| TEXAS INSTRUMENTS INCORPORATED
| Standard Linear and Logic Group
| IBIS Model of SN74ALVC245
| OCTAL BUS TRANSCEIVER WITH 3-STATE OUTPUTS
| This file contains package information for the following:
|  TVSOP 20-pin (DGV) package as [Component] ALVC245_DGV
|  SOIC 20-pin (DW) package as [Component] ALVC245_DW
|  SOP 20-pin (NS) package as [Component] ALVC245_NS
|  TSSOP 20-pin (PW) package as [Component] ALVC245_PW
|  QFN 20-pin (RGY) package as [Component] ALVC245_RGY
| This device can be powered at the following Vccs:
|  1.8 volt Vcc
|  2.5 volt Vcc
|  3.3 volt Vcc
| This file provides unique models under the [Model Selector] for each Vcc.
| For operation at a specific Vcc, select the appropriate model after each
| [Model Selector] keyword.
[IBIS Ver]   3.2
[Comment char]  |_char
[File Name]   sn74alvc245.ibs
[File Rev]   1.2 | d_die
[Date]   September 17, 2003
[Source]   Data created from TI-SPICE simulations at TI-SLL.
[Notes]   The following is an IBIS list for the SN74ALVC245.
   Please contact sllibis@ti.com with questions and
   comments concerning SLL IBIS models.
   - We removed Power_Clamp curve from the input models
   since there is no power clamp diode there.
   - Non-monotonic data in pulldown due to device characteristics.
[Disclaimer] Property of Texas Instruments Incorporated.  Unauthorized
   reproduction and/or distribution is strictly prohibited.
   This product is protected under copyright law.
   Created  2002, (C) Copyright  2002, Texas Instruments
   Incorporated, All Rights Reserved
   UNLESS THERE IS A SIGNED, WRITTEN AGREEMENT TO THE
   CONTRARY, TEXAS INSTRUMENTS (TI) IS PROVIDING THE IBIS
   MODELS  AND WITHOUT ANY WARRANTY, EXPRESSED OR
   IMPLIED.  TI assumes no liability for:
   1) the accuracy of the IBIS models provided to your
   company;
   2) the proper functioning of these IBIS Models in your
   design or for any resulting applications; or
   3) infringement of patents, copyrights or intellectual
   property rights resulting from your use of these IBIS
   models.
   TI provides IBIS Models as a service to our customers.
   You and your company shall not distribute, sell or give
   these models to anyone else without prior written
   permission from TI.
   TI reserves the right to make changes to our products or
   to discontinue any semiconductor product or service
   without notice, and advises our customers to obtain the
   latest version of relevant information to verify, before
   placing orders, that the information being relied on is
   current.
   Please be aware that your receipt and use of the IBIS
   information provided shall serve as acceptance of these
   terms and conditions.  If you do not accept these terms,
   you should return or destroy the IBIS models and any
   other accompanying information immediately.
| Component ALVC245_DGV 20-pin TVSOP
[Component]   ALVC245_DGV
[Manufacturer]  Texas Instruments, Inc.
[Package]
|   typ   min   max
R_pkg   4.400e-02   3.800e-02   4.800e-02
L_pkg   2.561e-09   2.236e-09   2.961e-09
C_pkg   3.420e-13   2.640e-13   4.460e-13
[Pin]   signal_name   model_name   R_pin   L_pin   C_pin
1   DIR   ALVC245_DIR   4.400e-02   2.935e-09   4.170e-13
2   A1   ALVC245_IO   4.200e-02   2.869e-09   4.460e-13
3   A2   ALVC245_IO   4.300e-02   2.399e-09   3.160e-13
4   A3   ALVC245_IO   4.400e-02   2.236e-09   2.650e-13
5   A4   ALVC245_IO   4.600e-02   2.278e-09   2.640e-13
6   A5   ALVC245_IO   4.500e-02   2.274e-09   2.640e-13
7   A6   ALVC245_IO   4.400e-02   2.285e-09   2.690e-13
8   A7   ALVC245_IO   4.300e-02   2.452e-09   3.200e-13
9   A8   ALVC245_IO   4.400e-02   2.900e-09   4.460e-13
10   GND   GND   4.400e-02   2.961e-09   4.180e-13
11   B8   ALVC245_IO   4.500e-02   2.954e-09   4.180e-13
12   B7   ALVC245_IO   4.200e-02   2.847e-09   4.430e-13
13   B6   ALVC245_IO   4.500e-02   2.453e-09   3.190e-13
14   B5   ALVC245_IO   4.500e-02   2.297e-09   2.690e-13
15   B4   ALVC245_IO   4.800e-02   2.334e-09   2.680e-13
16   B3   ALVC245_IO   4.800e-02   2.335e-09   2.670e-13
17   B2   ALVC245_IO   4.600e-02   2.299e-09   2.680e-13
18   B1   ALVC245_IO   4.600e-02   2.457e-09   3.200e-13
19   NOE   ALVC245_OE   4.300e-02   2.848e-09   4.410e-13
20   VCC   POWER   3.800e-02   2.812e-09   4.080e-13
| Component ALVC245_DW 20-pin SOIC
[Component]   ALVC245_DW
[Manufacturer]  Texas Instruments, Inc.
[Package]
|   typ   min   max
R_pkg   3.800e-02   3.300e-02   4.500e-02
L_pkg   5.012e-09   4.110e-09   6.349e-09
C_pkg   7.170e-13   5.300e-13   8.680e-13
[Pin]   signal_name   model_name   R_pin   L_pin   C_pin
1   DIR   ALVC245_DIR   4.200e-02   6.336e-09   8.650e-13
2   A1   ALVC245_IO   4.300e-02   5.542e-09   8.670e-13
3   A2   ALVC245_IO   3.400e-02   4.714e-09   7.320e-13
4   A3   ALVC245_IO   3.400e-02   4.377e-09   5.910e-13
5   A4   ALVC245_IO   3.600e-02   4.130e-09   5.330e-13
6   A5   ALVC245_IO   3.500e-02   4.111e-09   5.300e-13
7   A6   ALVC245_IO   3.400e-02   4.284e-09   5.830e-13
8   A7   ALVC245_IO   3.400e-02   4.634e-09   7.260e-13
9   A8   ALVC245_IO   4.000e-02   5.518e-09   8.650e-13
10   GND   GND   4.300e-02   6.349e-09   8.660e-13
11   B8   ALVC245_IO   4.100e-02   6.281e-09   8.610e-13
12   B7   ALVC245_IO   4.500e-02   5.561e-09   8.680e-13
13   B6   ALVC245_IO   3.300e-02   4.778e-09   7.420e-13
14   B5   ALVC245_IO   3.500e-02   4.414e-09   5.960e-13
15   B4   ALVC245_IO   3.500e-02   4.110e-09   5.330e-13
16   B3   ALVC245_IO   3.600e-02   4.130e-09   5.330e-13
17   B2   ALVC245_IO   3.400e-02   4.377e-09   5.910e-13
18   B1   ALVC245_IO   3.400e-02   4.714e-09   7.310e-13
19   NOE   ALVC245_OE   4.300e-02   5.569e-09   8.680e-13
20   VCC   POWER   4.200e-02   6.308e-09   8.640e-13
| Component ALVC245_NS 20-pin SOP
[Component]   ALVC245_NS
[Manufacturer]  Texas Instruments, Inc.
[Package]
|   typ   min   max
R_pkg   4.400e-02   2.900e-02   5.800e-02
L_pkg   3.666e-09   2.317e-09   5.115e-09
C_pkg   5.480e-13   3.160e-13   7.250e-13
[Pin]   signal_name   model_name   R_pin   L_pin   C_pin
1   DIR   ALVC245_DIR   5.800e-02   5.115e-09   7.250e-13
2   A1   ALVC245_IO   5.300e-02   4.591e-09   7.240e-13
3   A2   ALVC245_IO   4.900e-02   3.754e-09   5.720e-13
4   A3   ALVC245_IO   2.900e-02   2.549e-09   3.880e-13
5   A4   ALVC245_IO   3.100e-02   2.317e-09   3.160e-13
6   A5   ALVC245_IO   3.100e-02   2.317e-09   3.160e-13
7   A6   ALVC245_IO   2.900e-02   2.556e-09   3.990e-13
8   A7   ALVC245_IO   4.900e-02   3.754e-09   5.790e-13
9   A8   ALVC245_IO   5.300e-02   4.591e-09   7.240e-13
10   GND   GND   5.800e-02   5.115e-09   7.250e-13
11   B8   ALVC245_IO   5.800e-02   5.115e-09   7.250e-13
12   B7   ALVC245_IO   5.300e-02   4.591e-09   7.240e-13
13   B6   ALVC245_IO   4.900e-02   3.754e-09   5.790e-13
14   B5   ALVC245_IO   2.900e-02   2.557e-09   3.990e-13
15   B4   ALVC245_IO   3.100e-02   2.317e-09   3.160e-13
16   B3   ALVC245_IO   3.100e-02   2.317e-09   3.160e-13
17   B2   ALVC245_IO   2.900e-02   2.557e-09   3.990e-13
18   B1   ALVC245_IO   4.900e-02   3.754e-09   5.790e-13
19   NOE   ALVC245_OE   5.300e-02   4.591e-09   7.240e-13
20   VCC   POWER   5.800e-02   5.115e-09   7.250e-13
| Component ALVC245_PW 20-pin TSSOP
[Component]   ALVC245_PW
[Manufacturer]  Texas Instruments, Inc.
[Package]
|   typ   min   max
R_pkg   5.000e-02   4.200e-02   6.000e-02
L_pkg   2.802e-09   2.248e-09   3.553e-09
C_pkg   3.170e-13   2.020e-13   4.430e-13
[Pin]   signal_name   model_name   R_pin   L_pin   C_pin
1   DIR   ALVC245_DIR   5.500e-02   3.461e-09   4.400e-13
2   A1   ALVC245_IO   5.500e-02   3.150e-09   4.010e-13
3   A2   ALVC245_IO   4.200e-02   2.619e-09   3.020e-13
4   A3   ALVC245_IO   4.500e-02   2.273e-09   2.020e-13
5   A4   ALVC245_IO   4.500e-02   2.248e-09   2.240e-13
6   A5   ALVC245_IO   4.500e-02   2.273e-09   2.260e-13
7   A6   ALVC245_IO   4.400e-02   2.323e-09   2.050e-13
8   A7   ALVC245_IO   4.600e-02   2.704e-09   3.070e-13
9   A8   ALVC245_IO   6.000e-02   3.265e-09   4.110e-13
10   GND   GND   5.700e-02   3.506e-09   4.360e-13
11   B8   ALVC245_IO   5.800e-02   3.553e-09   4.370e-13
12   B7   ALVC245_IO   5.800e-02   3.193e-09   4.050e-13
13   B6   ALVC245_IO   4.200e-02   2.704e-09   3.110e-13
14   B5   ALVC245_IO   4.600e-02   2.392e-09   2.100e-13
15   B4   ALVC245_IO   4.700e-02   2.334e-09   2.290e-13
16   B3   ALVC245_IO   4.700e-02   2.300e-09   2.270e-13
17   B2   ALVC245_IO   4.700e-02   2.349e-09   2.070e-13
18   B1   ALVC245_IO   4.500e-02   2.677e-09   3.060e-13
19   NOE   ALVC245_OE   6.000e-02   3.235e-09   4.060e-13
20   VCC   POWER   5.600e-02   3.487e-09   4.430e-13
| Component ALVC245_RGY 20-pin QFN
[Component]   ALVC245_RGY
[Manufacturer]   Texas Instruments, Inc.
[Package]
|   typ   min   max
R_pkg   0.046   0.035   0.058
L_pkg   1.131nH   0.880nH   1.396nH
C_pkg   0.165pF   0.142pF   0.175pF
[Pin]   signal_name   model_name   R_pin   L_pin   C_pin
1   DIR   ALVC245_DIR   0.053   1.289nH   0.142pF
2   A1   ALVC245_IO   0.058   1.386nH   0.172pF
3   A2   ALVC245_IO   0.046   1.111nH   0.173pF
4   A3   ALVC245_IO   0.039   0.965nH   0.161pF
5   A4   ALVC245_IO   0.035   0.881nH   0.165pF
6   A5   ALVC245_IO   0.035   0.880nH   0.165pF
7   A6   ALVC245_IO   0.039   0.961nH   0.161pF
8   A7   ALVC245_IO   0.045   1.105nH   0.172pF
9   A8   ALVC245_IO   0.058   1.386nH   0.172pF
10   GND   GND   0.056   1.352nH   0.159pF
11   B8   ALVC245_IO   0.053   1.287nH   0.155pF
12   B7   ALVC245_IO   0.058   1.396nH   0.172pF
13   B6   ALVC245_IO   0.047   1.129nH   0.175pF
14   B5   ALVC245_IO   0.040   0.976nH   0.164pF
15   B4   ALVC245_IO   0.035   0.884nH   0.169pF
16   B3   ALVC245_IO   0.035   0.881nH   0.168pF
17   B2   ALVC245_IO   0.039   0.967nH   0.162pF
18   B1   ALVC245_IO   0.046   1.118nH   0.174pF
19   NOE   ALVC245_NOE   0.058   1.396nH   0.175pF
20   VCC   POWER   0.052   1.276nH   0.144pF
| Model ALVC245_OE
[Model Selector]   ALVC245_OE
ALVC245_OE_18   1.8 volt Vcc
ALVC245_OE_25   2.5 volt Vcc
ALVC245_OE_33   3.3 volt Vcc
| Model ALVC245_DIR
[Model Selector]   ALVC245_DIR
ALVC245_DIR_18   1.8 volt Vcc
ALVC245_DIR_25   2.5 volt Vcc
ALVC245_DIR_33   3.3 volt Vcc
| Model ALVC245_IO
[Model Selector]   ALVC245_IO
ALVC245_IO_18   1.8 volt Vcc
ALVC245_IO_25   2.5 volt Vcc
ALVC245_IO_33   3.3 volt Vcc
| Models and submodels in the file (9): ALVC245_OE_18 (Input), ALVC245_OE_25 (Input), ALVC245_OE_33 (Input), ALVC245_DIR_18 (Input), ALVC245_DIR_25 (Input), ALVC245_DIR_33 (Input), ALVC245_IO_18 (I/O), ALVC245_IO_25 (I/O), ALVC245_IO_33 (I/O)
